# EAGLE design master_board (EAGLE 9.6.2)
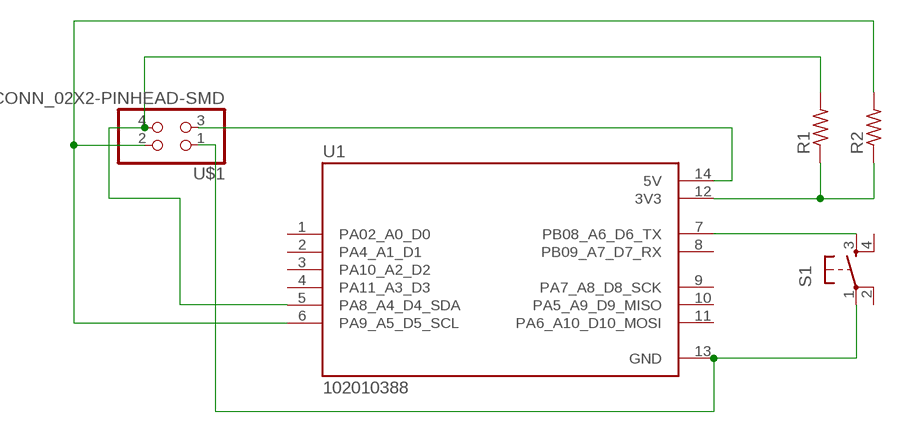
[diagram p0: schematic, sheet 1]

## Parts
R1  R1206FAB  [R1206FAB]
R2  R1206FAB  [R1206FAB]
S1  SW_SWITCH_TACTILE_6MM6MM_SWITCH  [6MM_SWITCH]
U1  102010388  [MODULE_102010388]
U$1  CONN_02X2-PINHEAD-SMD  [2X02SMD]

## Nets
N$1: R1.1 R2.1 U1.12(3V3)
N$2: R2.2 U1.6(PA9_A5_D5_SCL) U$1.2
N$3: R1.2 U1.5(PA8_A4_D4_SDA) U$1.4
N$6: U1.14(5V) U$1.3
N$7: S1.1(P) U1.13(GND) U$1.1
N$8: S1.3(S) U1.7(PB08_A6_D6_TX)
Unconnected: S1.2(P1) S1.4(S1) U1.1(PA02_A0_D0) U1.2(PA4_A1_D1) U1.3(PA10_A2_D2) U1.4(PA11_A3_D3) U1.8(PB09_A7_D7_RX) U1.9(PA7_A8_D8_SCK) U1.10(PA5_A9_D9_MISO) U1.11(PA6_A10_D10_MOSI)

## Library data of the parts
R1 R2 = fab-emma-re8nowiwt7yj8fhybscymuq61o:R: Resistor (US Symbol)
S1 = fab-emma-re8nowiwt7yj8fhybscymuq61o:SW_SWITCH_TACTILE_6MM: OMRON SWITCH
U1 = seeed:102010388: Check availability; AVAILABILITY: In Stock; DESCRIPTION: SAMD21G18 Seeeduino XIAO series ARM® Cortex®-M0 MCU 32-Bit Embedded Evaluation Board; MF: Seeed Technology Co., Ltd; MP: 102010388; PACKAGE: None; PRICE: None; PURCHASE-URL: https://pricing.snapeda.com/search/part/102010388/?ref=eda
U$1 = fab-emma-re8nowiwt7yj8fhybscymuq61o:CONN_02X2-PINHEAD-SMD

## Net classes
0 default: width 0.4 mm, drill 0.4 mm, clearance 0.4 mm

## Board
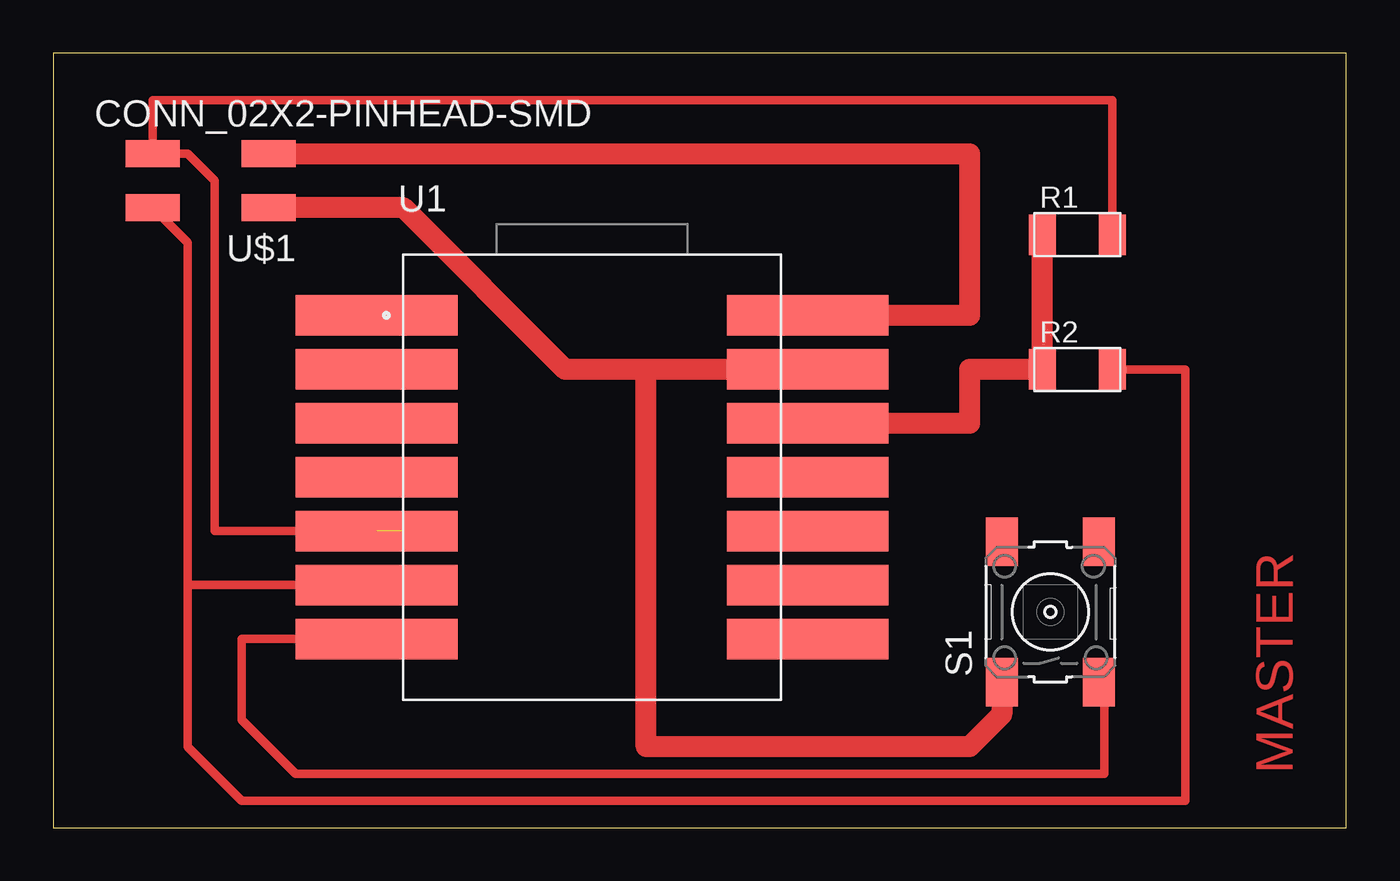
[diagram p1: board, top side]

Size 60.94 x 36.5 mm. Coordinates in mm from the lower left corner, seen from the top.
Outline: 0,0 60.94,0 60.94,36.5 0,36.5 0,0
Copper layers (1*16): Top 0.035mm / dielectric 1.5mm / Bottom 0.035mm
Design rules "default *": minimum track width 6mil, minimum drill 0.35mm, track to track 0.4mm, track to pad 0.4mm, pad to pad 0.4mm, via to via 0.4mm, smd to smd 0.4mm, copper to edge 40mil, drill to drill 6mil, minimum pad ring 10mil, minimum via ring 8mil, stop-mask expansion 4mil, vias tented up to drill 0mil, thermal gap 10mil

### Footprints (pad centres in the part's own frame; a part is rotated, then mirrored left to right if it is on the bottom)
R1206FAB = smd 1.27 x 1.905: 1 -1.651,0; 2 1.651,0
6MM_SWITCH = smd 2.286 x 1.524: 1 -3.302,2.286; 2 3.302,2.286; 3 -3.302,-2.286; 4 3.302,-2.286
MODULE_102010388 = smd 7.62 x 1.905: 1 -10.16,7.62; 2 -10.16,5.08; 3 -10.16,2.54; 4 -10.16,0; 5 -10.16,-2.54; 6 -10.16,-5.08; 7 -10.16,-7.62; 8 10.16,-7.62; 9 10.16,-5.08; 10 10.16,-2.54; 11 10.16,0; 12 10.16,2.54; 13 10.16,5.08; 14 10.16,7.62
2X02SMD = smd 2.54 x 1.27: 1 -2.54,1.27; 2 2.92,1.27; 3 -2.54,-1.27; 4 2.92,-1.27

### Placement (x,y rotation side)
R1  48.26,27.94 0 top
R2  48.26,21.59 0 top
S1  46.99,10.16 90 top
U1  25.4,16.51 0 top
U$1  7.62,30.48 180 top

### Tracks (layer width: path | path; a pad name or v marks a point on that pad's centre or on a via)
N$1
  Top 1: R1.1 R2.1 43.18,21.59 43.18,19.05 U1.12
N$2
  Top 0.4: U$1.2 6.35,27.56 6.35,11.43 | U1.6 6.35,11.43 | 6.35,11.43 6.35,3.81 8.89,1.27 53.34,1.27 53.34,21.59 R2.2
N$3  (1 unrouted)
  Top 0.4: R1.2 49.91,34.29 4.7,34.29 U$1.4 6.35,31.75 7.62,30.48 7.62,13.97 16.51,13.97
N$6
  Top 1: U$1.3 43.18,31.75 43.18,24.13 U1.14
N$7
  Top 1: U1.13 27.94,21.59 | 27.94,21.59 24.13,21.59 16.51,29.21 U$1.1 | S1.1 44.7,5.33 43.18,3.81 27.94,3.81 27.94,21.59
N$8
  Top 0.4: S1.3 49.53,6.6 49.53,2.54 11.43,2.54 8.89,5.08 8.89,8.89 U1.7

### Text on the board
Top: MASTER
